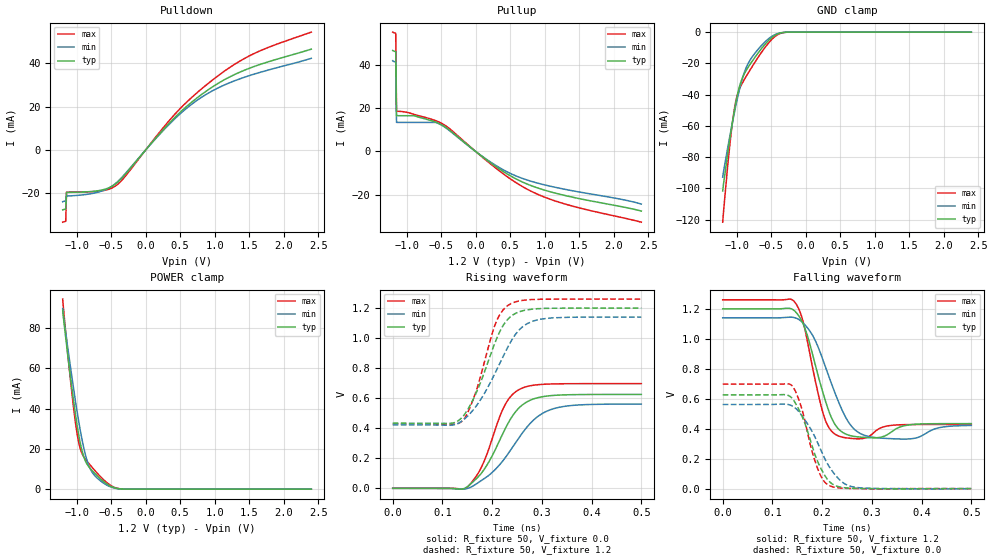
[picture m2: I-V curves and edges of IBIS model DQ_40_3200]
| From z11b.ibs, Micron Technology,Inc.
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| MODEL DQ_40_3200 (40 Ohm Data I/O with no ODT, 1600-3200Mbps)
[Model]   DQ_40_3200
Model_type   I/O
Vinl = 905.000mV
Vinh = 1015.000mV
Vmeas = 960.000mV
Vref = 1200.000mV
Cref = 0.0pF
Rref = 50.000Ohm
|   typ   min   max
|C_comp   0.780pF   0.730pF   0.830pF
C_comp_pullup   0.390pF   0.365pF   0.415pF
C_comp_pulldown   0.390pF   0.365pF   0.415pF
[Model Spec]
| Timing spec test load voltage corners
Vref   1.2000V   1.1400V   1.2600V
| Dynamic Overshoot Parameters from DDR4 Specification
|D_overshoot_ampl_h   0.40   NA   NA
|D_overshoot_ampl_l   0.40   NA   NA
|D_overshoot_area_h   0.0800n   NA   NA
|D_overshoot_area_l   0.0800n   NA   NA
[Voltage Range]   1.2000V   1.1400V   1.2600V
| Junction Temperature (Ambient temp is 35C typ, 95C min, 0C max)
[Temperature Range]   50.0   110.0   0.0
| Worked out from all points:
|   slope of the pulldown table from 0 to 0.18 V, typ, clamps not added: 27 ohm
|   slope of the pullup table from 0 to 0.18 V, typ, clamps not added: 41 ohm
|   GND clamp passes 1 mA (typ) near -0.39 V on its own axis
|   POWER clamp passes 1 mA (typ) near -0.48 V on its own axis
|   rising waveform, R_fixture 50, V_fixture 0.0: 20-80 % time 61.1ps typ, 79.3ps min, 48ps max; typ from 0 V to 0.625 V
|   rising waveform, R_fixture 50, V_fixture 1.2: 20-80 % time 54.7ps typ, 69.3ps min, 44.2ps max; typ from 0.434 V to 1.2 V
|   falling waveform, R_fixture 50, V_fixture 1.2: 20-80 % time 38.6ps typ, 49.7ps min, 31.4ps max; typ from 1.2 V to 0.434 V
|   falling waveform, R_fixture 50, V_fixture 0.0: 20-80 % time 41.8ps typ, 54ps min, 33.5ps max; typ from 0.625 V to 0 V
[Pulldown]
|   Voltage   I(typ)   I(min)   I(max)
-1.2V     -27.55mA   -23.81mA   -33.22mA
-1.156V   -27.16mA   -23.4mA    -32.8mA
-1.145V   -19.52mA   -21.17mA   -19.42mA
-687.3mV  -18.73mA   -19.4mA    -19mA
-545.5mV  -17.56mA   -17.71mA   -18.17mA
-414.5mV  -15.09mA   -14.82mA   -16.02mA
-305.5mV  -11.61mA   -11.26mA   -12.53mA
480mV     16.76mA    16.08mA    18.42mA
774.5mV   24.71mA    23.53mA    27.19mA
1.058V    30.86mA    28.74mA    34.4mA
1.625V    39.07mA    35.48mA    45.23mA
2.4V      46.45mA    42.25mA    54.32mA
[GND_clamp]
|   Voltage   I(typ)   I(min)   I(max)
-1.2V     -101.7mA   -92.86mA   -121.7mA
-1.135V   -79.96mA   -75.85mA   -88.92mA
-1.08V    -63.49mA   -62.76mA   -65.41mA
-1.036V   -51.56mA   -52.84mA   -50.65mA
-992.7mV  -41.38mA   -43.58mA   -41.02mA
-927.3mV  -30.76mA   -31.6mA    -33.57mA
-872.7mV  -25.55mA   -24.13mA   -29.29mA
-818.2mV  -21.61mA   -19.01mA   -25.29mA
-621.8mV  -9.659mA   -7.799mA   -11.96mA
-436.4mV  -1.919mA   -1.478mA   -2.611mA
-229.1mV  -17.2uA    -19.75uA   -20.83uA
2.4V      0A         0A         0A
[Pullup]
|   Voltage   I(typ)   I(min)   I(max)
-1.2V     46.58mA    41.86mA    55.08mA
-1.156V   46.03mA    41.25mA    54.5mA
-1.145V   16.48mA    13.4mA     18.54mA
-883.6mV  16.45mA    13.4mA     17.01mA
-567.3mV  13.38mA    13.3mA     14.07mA
-392.7mV  10.21mA    9.959mA    10.9mA
0V        727.4nA    681.7nA    814.1nA
316.4mV   -7.487mA   -6.918mA   -8.291mA
610.9mV   -13.1mA    -11.65mA   -14.92mA
883.6mV   -16.7mA    -14.5mA    -19.57mA
1.429V    -21.3mA    -18.31mA   -25.46mA
2.4V      -27.51mA   -24.29mA   -32.66mA
[Power Clamp]
|   Voltage   I(typ)   I(min)   I(max)
-1.2V     88.83mA    89.6mA     94.34mA
-1.135V   68.72mA    72.21mA    70.04mA
-1.058V   47.72mA    53.58mA    44.98mA
-1.004V   34.46mA    41.14mA    30.26mA
-960mV    25.46mA    31.98mA    21.99mA
-894.5mV  16.03mA    20.41mA    16.05mA
-807.3mV  10.5mA     10.53mA    12.15mA
-709.1mV  6.909mA    5.768mA    8.277mA
-545.5mV  2.223mA    1.735mA    2.842mA
-436.4mV  532.8uA    427.3uA    716.1uA
-294.5mV  16.22uA    18.62uA    20.69uA
2.4V      0A         0A         0A
[Ramp]
|   typ   min   max
dV/dt_r   375.12m/61.12p   336.65m/79.27p   418.24m/48.04p
dV/dt_f   459.72m/38.58p   431.14m/49.64p   499.21m/31.46p
R_load = 50
[Rising Waveform]
R_fixture = 50
V_fixture = 0.0
|   Time   V(typ)   V(min)   V(max)
0s        2.479uV    7.011uV    1.422uV
149ps     8.224mV    -2.065mV   5.284mV
180ps     107.8mV    55.29mV    152mV
199ps     209.2mV    102.4mV    318.9mV
227ps     401.7mV    206.8mV    562.3mV
242ps     487.1mV    278.8mV    628.2mV
260ps     553.1mV    365mV      666.7mV
293ps     604.5mV    481.1mV    690.2mV
329ps     619.9mV    535.2mV    695.6mV
500ps     625.2mV    561.1mV    697.1mV
[Rising Waveform]
R_fixture   = 50
V_fixture   = 1.2
V_fixture_min = 1.14
V_fixture_max = 1.26
|   Time   V(typ)   V(min)   V(max)
0s        433.8mV    422.3mV    428mV
116ps     432.6mV    419.9mV    426.6mV
141ps     477.8mV    452.3mV    451.6mV
167ps     628.2mV    543.3mV    639.1mV
207ps     979.9mV    774.3mV    1.099V
221ps     1.079V     870.8mV    1.184V
238ps     1.145V     979mV      1.23V
265ps     1.185V     1.085V     1.253V
299ps     1.197V     1.127V     1.259V
500ps     1.2V       1.14V      1.26V
[Falling Waveform]
R_fixture   = 50
V_fixture   = 1.2
V_fixture_min = 1.14
V_fixture_max = 1.26
|   Time   V(typ)   V(min)   V(max)
0s        1.2V       1.14V      1.26V
143ps     1.19V      1.142V     1.252V
162ps     1.097V     1.105V     1.11V
184ps     853.5mV    1.003V     754.3mV
204ps     613mV      836.9mV    479.2mV
230ps     408.9mV    602.8mV    355.4mV
259ps     351.8mV    416.4mV    334.8mV
296ps     339.4mV    346mV      352.2mV
339ps     377.5mV    333.1mV    422mV
500ps     433.8mV    421.4mV    428mV
[Falling Waveform]
R_fixture = 50
V_fixture = 0.0
|   Time   V(typ)   V(min)   V(max)
0s        625.2mV    561.3mV    697.1mV
139ps     604.5mV    553mV      688.2mV
158ps     494.6mV    492.9mV    545.1mV
178ps     302mV      392mV      268.6mV
191ps     180.2mV    305mV      132.9mV
203ps     100.5mV    215mV      52.5mV
216ps     42.24mV    137.2mV    17.73mV
241ps     7.526mV    41.6mV     2.746mV
267ps     1.568mV    8.69mV     600.5uV
500ps     7.719uV    -192.2uV   6.892uV
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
